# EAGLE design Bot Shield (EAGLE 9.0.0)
COMPANY: ADAFRUIT INDUSTRIES; DRAWN: KTOWN; REV: B
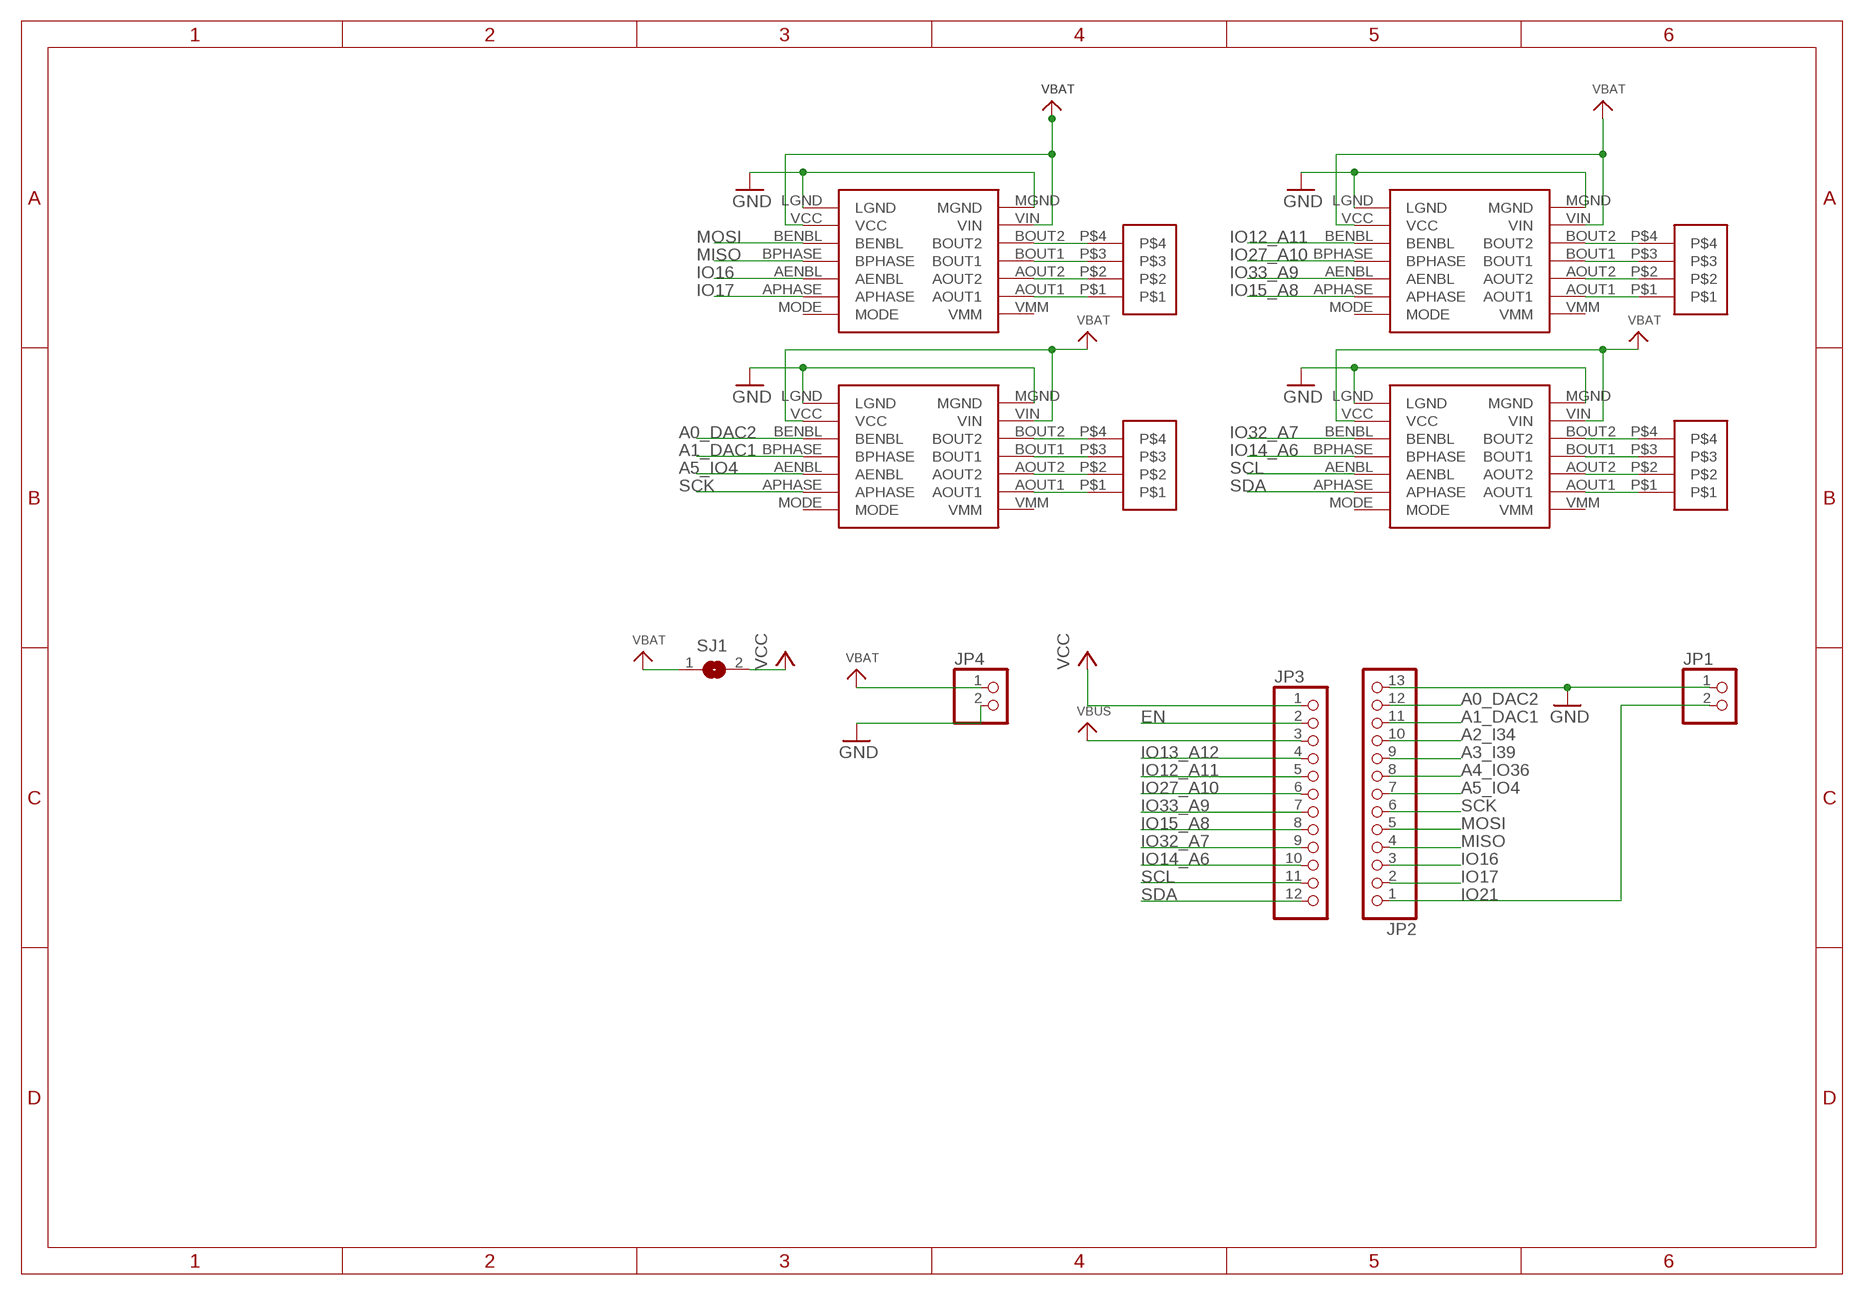
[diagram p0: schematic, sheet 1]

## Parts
JP1  PINHD-1X2  [1X02]
JP2  MICROBUILDER_HEADER-1X1313_PIN  [MICROBUILDER_1X13_ROUND_MIN]
JP3  HEADER-1X12_MIN  [1X12_ROUND_MIN]
JP4  PINHD-1X2  [1X02]
SJ1  SJ  [SJ]
U2  POLOLU_MOTOR_DRV8835FLOAT  [POLOLU_MOTOR_DRV_DRV8835_PAD_FLOAT]
U4  POLOLU_MOTOR_DRV8835FLOAT  [POLOLU_MOTOR_DRV_DRV8835_PAD_FLOAT]
U$1  POLOLU_MOTOR_DRV8835FLOAT  [POLOLU_MOTOR_DRV_DRV8835_PAD_FLOAT]
U$3  POLOLU_MOTOR_DRV8835FLOAT  [POLOLU_MOTOR_DRV_DRV8835_PAD_FLOAT]
U$10  4-HEADER  [4-HEADER]
U$11  4-HEADER  [4-HEADER]
U$12  4-HEADER  [4-HEADER]
U$13  4-HEADER  [4-HEADER]

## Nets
A0_DAC2: JP2.12 U$1.BENBL
A1_DAC1: JP2.11 U$1.BPHASE
A2_I34: JP2.10
A3_I39: JP2.9
A4_IO36: JP2.8
A5_IO4: JP2.7 U$1.AENBL
EN: JP3.2
GND: JP1.1 JP2.13 JP4.2 U2.LGND U2.MGND U4.LGND U4.MGND U$1.LGND U$1.MGND U$3.LGND U$3.MGND
IO12_A11: JP3.5 U$3.BENBL
IO13_A12: JP3.4
IO14_A6: JP3.10 U4.BPHASE
IO15_A8: JP3.8 U$3.APHASE
IO16: JP2.3 U2.AENBL
IO17: JP2.2 U2.APHASE
IO21: JP1.2 JP2.1
IO27_A10: JP3.6 U$3.BPHASE
IO32_A7: JP3.9 U4.BENBL
IO33_A9: JP3.7 U$3.AENBL
MISO: JP2.4 U2.BPHASE
MOSI: JP2.5 U2.BENBL
N$1 [pwr]: U2.BOUT2 U$10.P$4
N$2 [pwr]: U2.BOUT1 U$10.P$3
N$3 [pwr]: U2.AOUT2 U$10.P$2
N$4 [pwr]: U2.AOUT1 U$10.P$1
N$5 [pwr]: U$1.BOUT2 U$11.P$4
N$6 [pwr]: U$1.BOUT1 U$11.P$3
N$7 [pwr]: U$1.AOUT2 U$11.P$2
N$8 [pwr]: U$1.AOUT1 U$11.P$1
N$9 [pwr]: U$3.BOUT2 U$13.P$4
N$10 [pwr]: U$3.BOUT1 U$13.P$3
N$11 [pwr]: U$3.AOUT2 U$13.P$2
N$12 [pwr]: U$3.AOUT1 U$13.P$1
N$13 [pwr]: U4.BOUT2 U$12.P$4
N$14 [pwr]: U4.BOUT1 U$12.P$3
N$15 [pwr]: U4.AOUT2 U$12.P$2
N$16 [pwr]: U4.AOUT1 U$12.P$1
SCK: JP2.6 U$1.APHASE
SCL: JP3.11 U4.AENBL
SDA: JP3.12 U4.APHASE
VBAT [pwr]: JP4.1 SJ1.1 U2.VCC U2.VIN U4.VCC U4.VIN U$1.VCC U$1.VIN U$3.VCC U$3.VIN
VBUS: JP3.3
VCC: JP3.1 SJ1.2
Unconnected: U2.MODE U2.VMM U4.MODE U4.VMM U$1.MODE U$1.VMM U$3.MODE U$3.VMM

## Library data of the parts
JP1 JP4 = pinhead:PINHD-1X2: PIN HEADER
JP2 = Adafruit HUZZAH32 ESP32 Feather:MICROBUILDER_HEADER-1X13: PIN HEADER
JP3 = microbuilder:HEADER-1X12
SJ1 = jumper:SJ: SMD solder JUMPER
U2 U4 U$1 U$3 = pololu:POLOLU_MOTOR_DRV8835
U$10-U$13 = header:4-HEADER

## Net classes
0 default: width 0.254 mm
1 pwr: width 0.508 mm

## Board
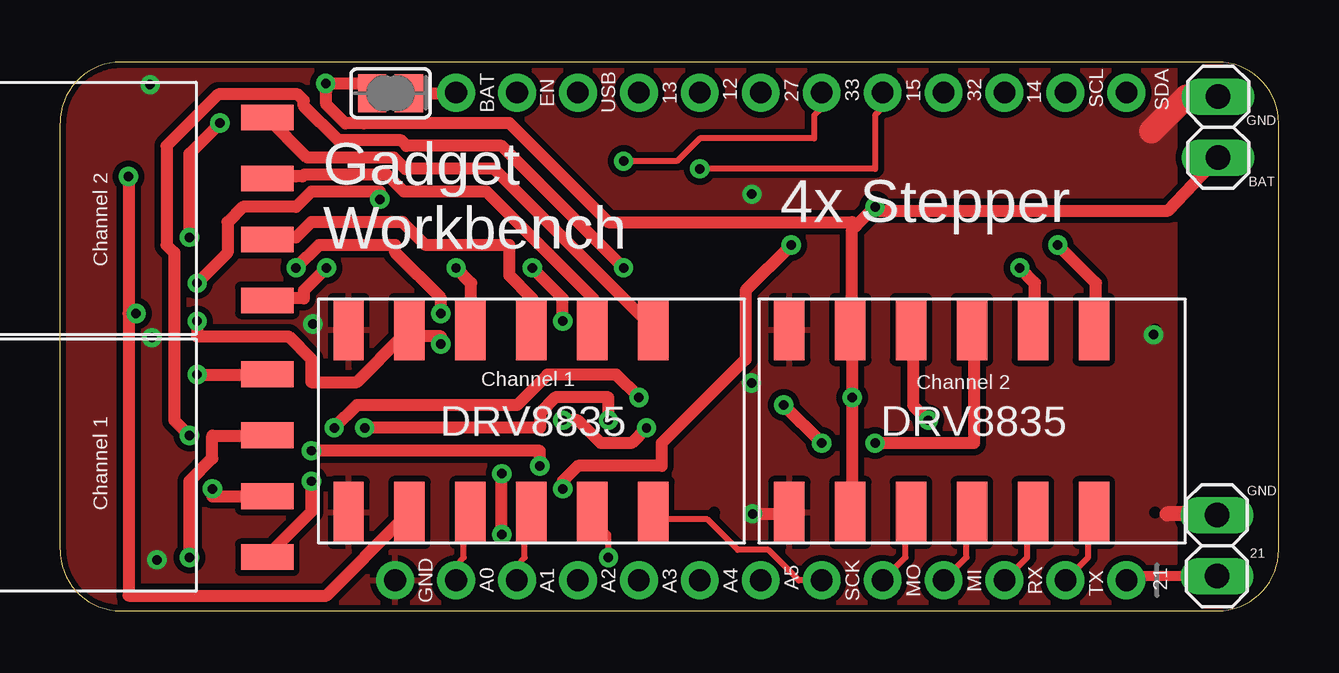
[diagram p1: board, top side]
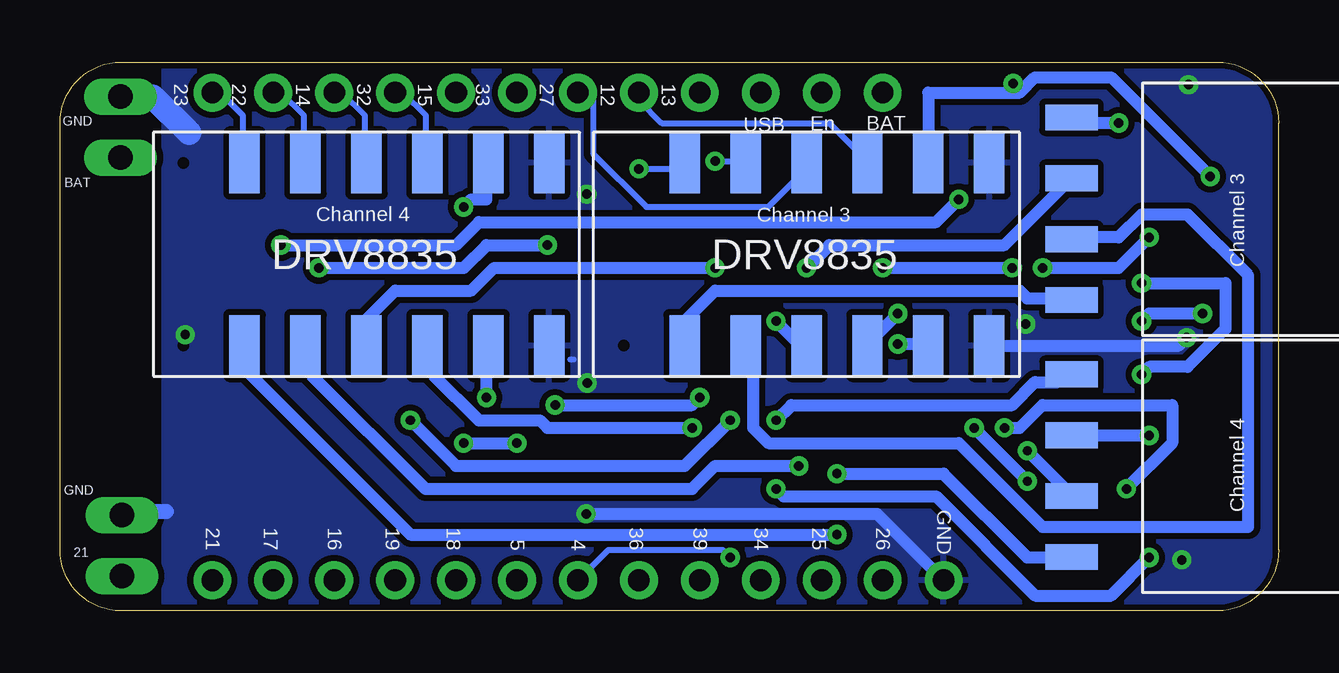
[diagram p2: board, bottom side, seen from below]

Size 50.8 x 22.86 mm. Coordinates in mm from the lower left corner, seen from the top.
Outline: 2.54,0 48.26,0 arc90 50.8,2.54 50.8,20.32 arc90 48.26,22.86 2.54,22.86 arc90 0,20.32 0,2.54 arc90 2.54,0
Copper layers (1*16): Top 0.035mm / dielectric 1.5mm / Bottom 0.035mm
Design rules "adafruit 7-7 *": minimum track width 6mil, minimum drill 15.5mil, track to track 8mil, track to pad 7mil, pad to pad 7mil, via to via 7mil, smd to smd 7mil, copper to edge 10mil, drill to drill 8mil, minimum pad ring 10mil, minimum via ring 8mil, stop-mask expansion 2mil, vias tented up to drill 20mil, thermal gap 10mil

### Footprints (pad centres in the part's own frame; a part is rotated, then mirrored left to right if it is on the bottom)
1X02 = drill 1.016 long: 1 -1.27,0; 2 1.27,0
MICROBUILDER_1X13_ROUND_MIN = drill 0.9 pad 1.575: 1 -19.05,0; 2 -16.51,0; 3 -13.97,0; 4 -11.43,0; 5 -8.89,0; 6 -6.35,0; 7 -3.81,0; 8 -1.27,0; 9 1.27,0; 10 3.81,0; 11 6.35,0; 12 8.89,0; 13 11.43,0
1X12_ROUND_MIN = drill 0.9 pad 1.575: 1 -13.97,0; 2 -11.43,0; 3 -8.89,0; 4 -6.35,0; 5 -3.81,0; 6 -1.27,0; 7 1.27,0; 8 3.81,0; 9 6.35,0; 10 8.89,0; 11 11.43,0; 12 13.97,0
SJ = smd 1.168 x 1.6: 1 -0.762,0; 2 0.762,0
POLOLU_MOTOR_DRV_DRV8835_PAD_FLOAT = smd 2.54 x 1.27: AENBL 1.27,6.35; AOUT1 8.89,3.81; AOUT2 8.89,6.35; APHASE 1.27,3.81; BENBL 1.27,11.43; BOUT1 8.89,8.89; BOUT2 8.89,11.43; BPHASE 1.27,8.89; LGND 1.27,16.51; MGND 8.89,16.51; VCC 1.27,13.97; VIN 8.89,13.97 | smd 0 x 0: MODE 1.27,1.27; VMM 8.89,1.27
4-HEADER = smd 2.184 x 1.067: P$1 0,0; P$2 0,-2.54; P$3 0,-5.08; P$4 0,-7.62

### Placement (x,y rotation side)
JP1  48.22,2.72 270 top
JP2  25.4,1.27 180 top
JP3  30.48,21.59 0 top
JP4  48.27,20.15 90 top
SJ1  13.78,21.56 0 top
U2  46.91,2.83 90 top
U4  46.91,19.93 270 bottom
U$1  28.54,2.83 90 top
U$3  28.57,19.93 270 bottom
U$10  8.64,9.85 0 top
U$11  8.64,20.55 0 top
U$12  8.64,2.24 180 bottom
U$13  8.64,12.94 180 bottom

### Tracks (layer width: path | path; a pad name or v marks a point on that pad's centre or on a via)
A0_DAC2
  Top 0.254: JP2.12 16.51,1.91 16.83,2.22 16.83,3.81 U$1.BENBL
A1_DAC1
  Top 0.254: JP2.11 19.05,1.91 19.37,2.22 19.37,3.81 U$1.BPHASE
A5_IO4  (via drill 0.39)
  Top 0.254: v22.86,2.22 22.86,3.17 22.23,3.81 U$1.AENBL
  Bottom 0.254: v22.86,2.22 23.18,2.54 27.94,2.54 JP2.7
GND  (via drill 0.39)
  Top 0.508: v28.87,4.04 30.34,4.04 U2.LGND
  Top 0.635: 48.17,4.04 46.14,4.04
  Top 1.016: JP4.2 46.94,21.43 45.49,19.98
  Bottom 0.254: 47.94,4.13 JP1.1 | 46.35,4.13 46.34,4.25 | 29.53,10.48 29.39,10.48
  Bottom 0.508: v28.87,4.04 16.74,4.04 JP2.13 | U$3.MGND 4.17,11.04 v3.83,11.38
  Bottom 0.635: 46.35,4.13 47.94,4.13
  Bottom 1.016: JP4.2 46.93,21.43 45.41,19.91
  other vias: 28.84,17.36 10.54,11.95 3.76,21.92 4.04,2.12 45.58,11.51 28.83,9.49
  pour Top (isolate 0.254): 0,22.86 46.45,22.86 46.45,0 0,0
  pour Bottom (isolate 0.254): 0,22.86 46.45,22.86 46.45,0 0,0
IO12_A11
  Bottom 0.254: JP3.5 26.67,21.27 25.72,20.32 18.73,20.32 17.14,18.73 U$3.BENBL
IO14_A6
  Bottom 0.254: JP3.10 39.05,21.59 38.1,20.64 38.1,18.73 U4.BPHASE
IO15_A8  (via drill 0.39)
  Top 0.254: v26.67,18.41 33.97,18.41 33.97,20.64 34.29,20.95 JP3.8
  Bottom 0.254: v26.67,18.41 24.77,18.41 U$3.APHASE
IO16
  Top 0.254: JP2.3 40.32,2.22 40.32,3.81 U2.AENBL
IO17
  Top 0.254: JP2.2 42.86,2.22 42.86,3.81 U2.APHASE
IO21
  Top 0.406: JP1.2 44.63,1.45 JP2.1
IO27_A10
  Bottom 0.254: JP3.6 28.57,21.59 28.57,19.05 26.35,16.83 21.27,16.83 19.68,18.41 U$3.BPHASE
IO32_A7
  Bottom 0.254: JP3.9 36.51,21.59 35.56,20.64 35.56,18.73 U4.BENBL
IO33_A9  (via drill 0.39)
  Top 0.254: v23.5,18.73 25.72,18.73 26.67,19.68 31.43,19.68 31.43,20.64 31.75,20.95 JP3.7
  Bottom 0.254: v23.5,18.73 22.23,18.73 U$3.AENBL
MISO
  Top 0.254: JP2.4 37.78,2.22 37.78,3.81 U2.BPHASE
MOSI
  Top 0.254: JP2.5 35.24,2.22 35.24,3.81 U2.BENBL
N$1  (via drill 0.39)
  Top 0.508: v10.48,5.4 10.48,4.13 8.89,2.54 U$10.P$4 | v12.7,7.62 20,7.62 20,8.26 20.64,8.89 22.86,8.89 v22.86,7.94 | v36.2,7.94 35.56,8.57 35.56,11.43 U2.BOUT2
  Bottom 0.508: v12.7,7.62 v10.48,5.4 | v22.86,7.94 24.77,6.03 34.29,6.03 v36.2,7.94
N$2  (via drill 0.39)
  Top 0.508: v6.35,5.08 6.35,4.76 8.57,4.76 U$10.P$3 | v11.43,7.62 12.38,8.57 19.05,8.57 20.32,9.84 23.18,9.84 v24.13,8.89 | v31.75,6.99 v30.16,8.57 | v33.97,6.99 38.1,6.99 38.1,11.43 U2.BOUT1
  Bottom 0.508: v6.35,5.08 4.45,6.99 4.45,8.57 9.84,8.57 10.79,7.62 v11.43,7.62 | v24.13,8.89 24.45,8.57 v30.16,8.57 | v33.97,6.99 v31.75,6.99
N$3  (via drill 0.39)
  Top 0.508: v5.4,2.22 5.4,5.4 6.35,6.35 6.35,7.3 8.57,7.3 U$10.P$2 | v20.95,5.08 20.95,5.4 21.59,6.03 25.08,6.03 25.08,6.99 28.57,10.48 28.57,13.34 v30.48,15.24 | v40.01,14.29 40.64,13.65 40.64,11.75 U2.AOUT2
  Bottom 0.508: v5.4,2.22 6.99,0.64 10.16,0.64 14.29,4.76 20.64,4.76 v20.95,5.08 | v30.48,15.24 33.02,15.24 33.97,14.29 v40.01,14.29
N$4  (via drill 0.39)
  Top 0.508: v5.71,9.84 8.57,9.84 U$10.P$1 | v5.71,13.65 6.99,14.92 6.99,16.19 7.62,16.83 9.84,16.83 10.48,17.46 13.34,17.46 v13.34,17.14 | v41.59,15.24 43.18,13.65 43.18,11.75 U2.AOUT1
  Bottom 0.508: v5.71,9.84 5.4,10.16 3.81,10.16 2.22,11.75 2.22,13.65 v5.71,13.65 | v13.34,17.14 14.29,16.19 33.34,16.19 34.29,15.24 v41.59,15.24
N$5  (via drill 0.39)
  Top 0.508: v11.11,14.29 10.16,13.34 10.16,13.02 8.89,13.02 U$11.P$4 | v16.51,14.29 17.14,13.65 17.14,11.75 U$1.BOUT2
  Bottom 0.508: v16.51,14.29 v11.11,14.29
N$6
  Top 0.508: U$11.P$3 8.89,15.56 9.84,15.56 10.48,16.19 14.29,16.19 15.24,15.24 18.73,15.24 18.73,13.97 19.68,13.02 19.68,11.75 U$1.BOUT1
N$7
  Top 0.508: U$11.P$2 8.89,18.1 9.31,18.1 9.84,18.1 10.11,18.1 10.18,18.17 13.63,18.17 14.34,17.46 17.78,17.46 22.23,13.02 22.23,11.75 U$1.AOUT2
N$8
  Top 0.508: 8.89,20.64 U$11.P$1 10.31,18.89 13.92,18.89 14.39,18.41 18.1,18.41 24.45,12.06 24.45,11.75 U$1.AOUT1
N$9  (via drill 0.39)
  Top 0.508: v6.67,20.32 5.4,19.05 v5.4,15.56 | v9.84,14.29 10.79,15.24 13.97,15.24 13.97,14.92 15.88,13.02 v15.88,12.38
  Bottom 0.508: v6.67,20.32 8.57,20.32 U$13.P$4 | v5.4,15.56 6.67,14.29 v9.84,14.29 | v15.88,12.38 17.14,11.11 U$3.BOUT2
N$10  (via drill 0.39)
  Top 0.508: v19.68,14.29 20.95,13.02 v20.95,12.06
  Bottom 0.508: v19.68,14.29 18.73,15.24 11.43,15.24 8.89,17.78 U$13.P$3 | v20.95,12.06 20,11.11 19.68,11.11 U$3.BOUT1
N$11
  Bottom 0.508: U$13.P$2 8.57,15.56 6.67,15.56 5.71,16.51 3.81,16.51 1.27,13.97 1.27,3.49 9.84,3.49 13.34,6.99 21.27,6.99 21.91,7.62 21.91,10.79 U$3.AOUT2
N$12
  Bottom 0.508: U$13.P$1 8.89,13.02 10.48,13.02 10.79,13.34 23.5,13.34 24.77,12.06 24.77,11.11 U$3.AOUT1
N$13  (via drill 0.39)
  Top 0.508: v20.95,7.94 21.59,7.94 22.54,6.99 23.81,6.99 v24.45,7.62
  Bottom 0.508: v20.95,7.94 20.32,8.57 11.11,8.57 10.16,9.53 9.21,9.53 8.89,9.84 U$12.P$4 | v24.45,7.62 30.48,7.62 30.8,7.94 33.34,7.94 35.24,9.84 35.24,10.79 U4.BOUT2
N$14  (via drill 0.39)
  Top 0.508: v5.4,7.3 4.76,7.94 4.76,14.92 4.45,15.24 4.45,19.37 6.6,21.52 9.91,21.52 10.17,21.27 10.17,21.02 11.6,19.6 14.22,19.6 14.45,19.37 18.41,19.37 v23.5,14.29
  Bottom 0.508: v5.4,7.3 8.57,7.3 U$12.P$3 | v23.5,14.29 32.7,14.29 33.66,13.34 36.83,13.34 38.1,12.06 38.1,11.11 U4.BOUT1
N$15  (via drill 0.39)
  Top 0.508: v10.48,6.67 20,6.67 v20,6.03
  Bottom 0.508: v10.48,6.67 8.89,5.08 U$12.P$2 | v20,6.03 23.5,6.03 24.45,5.08 35.56,5.08 40.32,9.84 40.32,10.79 U4.AOUT2
N$16  (via drill 0.39)
  Top 0.508: v18.41,3.17 v18.41,5.71
  Bottom 0.508: v18.41,5.71 13.97,5.71 10.48,2.22 8.89,2.22 U$12.P$1 | v18.41,3.17 36.2,3.17 42.86,9.84 42.86,10.79 U4.AOUT1
SCK
  Top 0.254: JP2.6 30.8,1.27 29.53,2.54 28.26,2.54 26.99,3.81 24.77,3.81 U$1.APHASE
SCL
  Bottom 0.254: JP3.11 41.59,21.59 40.64,20.64 40.64,18.73 U4.AENBL
SDA
  Bottom 0.254: JP3.12 44.13,21.59 43.18,20.64 43.18,18.73 U4.APHASE
VBAT  (via drill 0.39)
  Top 0.508: U2.VCC 33.02,4.13 v33.02,8.89 33.02,11.43 U2.VIN 33.02,11.75 33.02,15.88 33.18,16.03 | 33.18,16.03 v33.97,16.83 34.13,16.67 46.2,16.67 JP4.1 | v15.88,11.11 15.88,11.43 14.61,11.43 U$1.VIN 14.29,11.43 12.38,9.53 10.48,9.53 10.48,10.48 9.53,11.43 5.71,11.43 v5.71,12.06 | v2.86,18.1 2.86,12.38 | 2.86,12.38 2.86,0.64 11.11,0.64 14.29,3.81 U$1.VCC | 2.86,12.38 v3.17,12.38 | 33.18,16.03 33.02,16.19 22.86,16.19 18.73,20.32 12.68,20.32 12.66,20.31 11.89,20.31 11.1,21.1 11.1,21.66 11.07,21.68 v11.07,21.97 12.61,21.97 SJ1.1
  Bottom 0.508: v33.02,8.89 33.02,10.79 U4.VIN | v33.97,16.83 33.66,17.14 33.02,17.14 33.02,18.41 U4.VCC | v15.88,11.11 14.61,11.11 U$3.VIN | v2.86,18.1 6.99,22.23 10.16,22.23 10.79,21.59 | 10.79,21.59 14.61,21.59 14.61,18.73 U$3.VCC | v5.71,12.06 5.4,12.38 v3.17,12.38 | v11.07,21.97 10.79,21.69 10.79,21.59
VCC
  Top 0.508: SJ1.2 16.48,21.57 JP3.1

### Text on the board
tPlace: BAT | EN | USB | 13 | 12 | 27 | 33 | 15 | 32 | 14 | SCL | SDA | GND | BAT | 4x Stepper | Gadget / Workbench | Channel 2 | Channel 1 | Channel 2 | GND | Channel 1 | 21 | GND | A0 | A1 | A2 | A3 | A4 | A5 | SCK | MO | MI | RX | TX | 21
bPlace: 13 | 12 | 27 | 33 | 15 | 32 | 14 | 22 | 23 | BAT | En | USB | GND | BAT | Channel 3 | Channel 4 | Channel 3 | GND | Channel 4 | GND | 26 | 25 | 34 | 39 | 36 | 4 | 5 | 18 | 19 | 16 | 17 | 21 | 21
